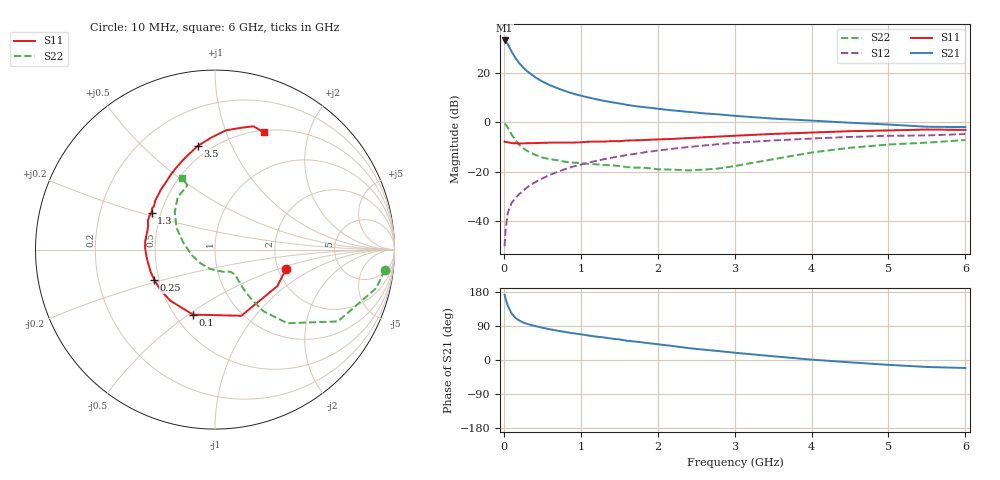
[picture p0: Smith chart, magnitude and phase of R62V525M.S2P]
! SIEMENS Small Signal Semiconductors
! BFR193
! Si NPN RF Bipolar Junction Transistor in SOT23
! VCE = 2.5 V  IC = 25 mA
! Common Emitter S-Parameters:  May  1996
# GHz  S  MA  R  50
!  f  S11  S21  S12  S22
! GHz  MAG  ANG  MAG  ANG  MAG  ANG  MAG  ANG
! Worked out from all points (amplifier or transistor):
!   36 points, 10 MHz to 6 GHz, reference 50 ohm
!   highest |S21| = 33.3 dB at 10 MHz (marker M1)
!   |S21| within 3 dB of that: start of sweep to 75.22 MHz
!   unconditionally stable (mu >= 1): 484.9 MHz to 1.875 GHz
!   at 250 MHz: K = 0.88, MSG = 25.0 dB, |S12| = -27.7 dB
!   at 1.4 GHz: K = 1.02, MAG = 10.5 dB, |S12| = -14.3 dB
!   at 6 GHz: K = 0.95, MSG = 1.4 dB, |S12| = -4.7 dB
!   S11 on the Smith chart (normalised r, x): 10 MHz: 2.20, -0.58; 100 MHz: 0.61, -0.52; 250 MHz: 0.47, -0.18; 1.3 GHz: 0.44, +0.22; 3.5 GHz: 0.43, +0.75; 6 GHz: 0.52, +1.37
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0.01  0.4097 -15.5  46.11 171.7  0.0031 84.5  0.9539 -6.8
0.02  0.4025 -30.3  45.06 163.6  0.006 81.4  0.9228 -13.5
0.05  0.3968 -68.3  38.78 143.8  0.0144 70.6  0.7932 -30.3
0.1  0.3825 -108.7  27.56 123.3  0.0232 64.7  0.575 -45.5
0.15  0.3784 -131.4  20.43 111.3  0.0293 64.5  0.4369 -51.8
0.2  0.3777 -144.3  16.04 104.3  0.0354 65.6  0.3551 -53.5
0.25  0.3775 -153.6  13.08 99.1  0.041 66.6  0.3015 -54.1
0.3  0.3793 -160.5  11.05 95.4  0.0479 68.4  0.2671 -53.9
0.4  0.3813 -170.2  8.437 90.0  0.0606 69.7  0.2234 -53.1
0.5  0.386 -177.1  6.773 85.2  0.0733 70.6  0.1944 -52.1
0.6  0.3901 177.6  5.693 81.0  0.0868 70.3  0.18 -52.0
0.8  0.3902 168.1  4.321 73.9  0.1135 69.3  0.1594 -53.3
0.9  0.3912 163.7  3.858 70.5  0.1273 68.6  0.154 -54.7
1.1  0.407 156.7  3.213 64.6  0.1532 66.7  0.1447 -58.2
1.3  0.4091 149.8  2.748 59.5  0.1798 64.2  0.137 -63.3
1.6  0.4298 141.0  2.28 50.9  0.2186 60.5  0.1247 -75.3
2.2  0.4649 125.8  1.755 36.8  0.2942 52.1  0.1105 -104.8
2.6  0.501 116.3  1.532 27.3  0.3411 46.0  0.1106 -134.5
3.5  0.5861 99.4  1.199 9.9  0.4319 31.9  0.1795 168.1
4.5  0.6665 84.9  0.989 -6.1  0.5091 17.7  0.307 136.9
5.5  0.7198 72.7  0.82 -18.4  0.5467 3.5  0.3904 113.2
6  0.7074 67.3  0.806 -21.1  0.5827 -0.6  0.4412 114.8
